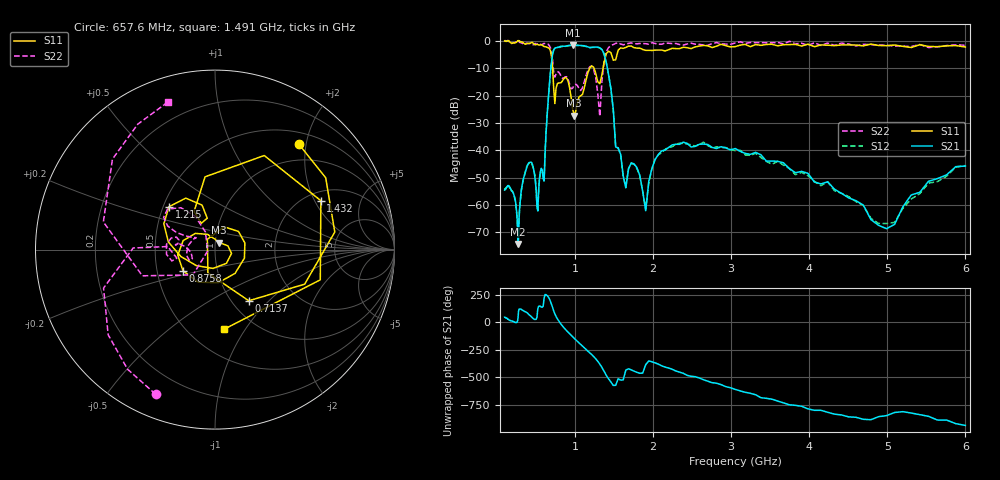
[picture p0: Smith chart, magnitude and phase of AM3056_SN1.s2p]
# Hz S DB R 50
!freq MagS11 AngS11 MagS21 AngS21 MagS12 AngS12 MagS22 AngS22
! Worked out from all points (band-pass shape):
!   201 points, 100 MHz to 6 GHz, reference 50 ohm
!   highest |S21| = -1.53 dB at 970.2 MHz (marker M1); lowest = -74.3 dB at 272.7 MHz (marker M2)
!   |S21| within 3 dB of the highest: 717.6 MHz to 1.371 GHz (653.4 MHz wide, 62.6 % of centre)
!   lowest |S11| = -27.4 dB at 990.3 MHz (marker M3), VSWR 1.09, Z = 51.9 + j3.96 ohm
!   |S11| at or under -10 dB: 714.9 MHz to 1.189 GHz (474.5 MHz wide, 49.8 % of centre); 1.245 GHz to 1.36 GHz (115.6 MHz wide, 8.88 % of centre)
!   |S22| runs from -27.6 to 0.2 dB; largest |S21 - S12| = 0.49
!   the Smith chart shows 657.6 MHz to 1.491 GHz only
!   S11 on the Smith chart (normalised r, x): 657.6 MHz: 0.70, +1.87; 713.7 MHz: 1.19, -0.77; 875.8 MHz: 0.68, -0.17; 1.215 GHz: 0.54, +0.29; 1.432 GHz: 2.38, +2.25; 1.491 GHz: 0.73, -0.81
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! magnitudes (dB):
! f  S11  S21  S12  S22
! 100 MHz  0.0  -54.6  -54.4  0.2
! 272.7 MHz  0.1  -74.3  -75.1  0.1
! 378.4 MHz  -1.1  -46.7  -46.3  -0.8
! 525 MHz  -1.3  -62.2  -62.1  -1.1
! 605.9 MHz  -2.0  -51.3  -50.9  -0.9
! 657.6 MHz  -2.5  -21.9  -21.9  -1.2
! 713.7 MHz  -9.3  -5.0  -4.8  -6.8
! 875.8 MHz  -13.4  -2.0  -2.0  -13.1
! 970.2 MHz  -24.7  -1.5  -1.6  -17.3
! 990.3 MHz  -27.4  -1.5  -1.7  -16.2
! 1.097 GHz  -19.5  -1.7  -1.7  -17.2
! 1.215 GHz  -9.1  -2.4  -2.3  -9.2
! 1.319 GHz  -15.6  -2.5  -2.5  -27.6
! 1.432 GHz  -3.7  -12.5  -12.2  -2.4
! 1.491 GHz  -7.0  -24.9  -25.4  -1.3
! 1.652 GHz  -2.4  -53.8  -53.6  -1.2
! 1.907 GHz  -3.4  -62.2  -61.5  -1.0
! 2.069 GHz  -3.3  -41.5  -41.6  -1.2
! 3.053 GHz  -2.1  -39.4  -40.2  -0.7
! 4.067 GHz  -2.1  -51.6  -51.4  -0.6
! 5.094 GHz  -1.5  -67.1  -66.4  -1.8
! 6 GHz  -2.2  -45.8  -45.6  -1.6
